[IBIS Ver]   3.2
[Comment Char]   |_char
[File Name]   sprm310.ibs
[File Rev]   1.0
[Date]   November 15, 2006
[Source]   From Ansoft Q3D ver 7.0 result.
[Notes]
[Disclaimer]
[Copyright]
[Component]   c2802ggm
[Manufacturer]   ti
[Package]
| variable   typ   min   max
R_pkg   2.43797e-001  1.95419e-001  3.27441e-001
L_pkg   3.68971n   2.87180n   5.33480n
C_pkg   0.700156p   0.378269p   1.23931p
[Pin]  signal_name   model_name   R_pin   L_pin   C_pin
B2   1   NC   2.35E-01   3.5513n   0.48473p
B1   2   NC   2.07E-01   3.0351n   0.467163p
C2   3   NC   2.47E-01   3.6211n   0.586473p
C3   4   NC   2.97E-01   4.5479n   0.708552p
C1   5   NC   2.19E-01   3.3047n   0.476389p
D2   6   NC   2.49E-01   3.6161n   0.555465p
D1   7   NC   2.15E-01   3.1776n   0.466284p
D3   8   NC   2.78E-01   4.1721n   0.675765p
E1   9   NC   2.16E-01   3.2216n   0.642896p
E2   10   NC   2.48E-01   3.6839n   0.861315p
E3   11   NC   2.90E-01   4.3193n   1.09313p
E4   12   NC   3.06E-01   4.8351n   1.23931p
E5   13   NC   3.27E-01   5.3348n   1.07834p
F1   14   NC   2.08E-01   3.0435n   0.550091p
F2   15   NC   2.37E-01   3.5019n   0.697553p
F3   16   NC   2.62E-01   4.1156n   1.04238p
F4   17   NC   2.93E-01   4.6685n   1.20271p
G4   18   NC   2.97E-01   4.7427n   1.03722p
G1   19   NC   2.03E-01   3.0288n   0.562932p
G2   20   NC   2.36E-01   3.4697n   0.651476p
G3   21   NC   2.72E-01   4.1098n   0.71232p
H1   22   NC   2.05E-01   3.0077n   0.489134p
H2   23   NC   2.38E-01   3.5337n   0.516547p
J1   24   NC   2.07E-01   3.0262n   0.418333p
K1   25   NC   2.15E-01   3.2729n   0.37954p
J2   26   NC   2.33E-01   3.5336n   0.483363p
K2   27   NC   2.03E-01   2.9784n   0.462757p
J3   28   NC   2.33E-01   3.4569n   0.577621p
H3   29   NC   2.71E-01   4.227n   0.695222p
K3   30   NC   1.95E-01   2.8906n   0.448812p
J4   31   NC   2.28E-01   3.374n   0.532016p
K4   32   NC   1.98E-01   2.8808n   0.454568p
H4   33   NC   2.65E-01   4.0698n   0.662835p
K5   34   NC   2.08E-01   3.1623n   0.638546p
J5   35   NC   2.46E-01   3.7519n   0.852293p
H5   36   NC   2.72E-01   4.2745n   1.07169p
G5   37   NC   2.97E-01   4.8506n   1.22295p
F5   38   NC   3.19E-01   5.2752n   1.05779p
K6   39   NC   2.07E-01   3.0553n   0.550089p
J6   40   NC   2.44E-01   3.6885n   0.755436p
H6   41   NC   2.74E-01   4.2729n   1.04565p
G6   42   NC   2.98E-01   4.6879n   1.20666p
G7   43   NC   3.08E-01   4.903n   1.03945p
K7   44   NC   2.10E-01   3.1053n   0.568618p
J7   45   NC   2.46E-01   3.6494n   0.659376p
H7   46   NC   2.88E-01   4.3538n   0.721025p
K8   47   NC   2.11E-01   3.1159n   0.491296p
J8   48   NC   2.47E-01   3.6522n   0.521398p
K9   49   NC   2.17E-01   3.2053n   0.425489p
K10   50   NC   2.14E-01   3.2751n   0.378399p
J9   51   NC   2.35E-01   3.5602n   0.485257p
J10   52   NC   2.07E-01   3.0498n   0.469529p
H9   53   NC   2.37E-01   3.5029n   0.580917p
H8   54   NC   2.75E-01   4.2366n   0.691548p
H10   55   NC   2.00E-01   2.9155n   0.45106p
G9   56   NC   2.36E-01   3.4315n   0.538278p
G10   57   NC   2.03E-01   2.922n   0.45761p
G8   58   NC   2.70E-01   4.1176n   0.665059p
F10   59   NC   2.11E-01   3.1329n   0.643673p
F9   60   NC   2.46E-01   3.6694n   0.861259p
F8   61   NC   2.69E-01   4.0897n   1.07509p
F7   62   NC   2.92E-01   4.5944n   1.22997p
F6   63   NC   3.16E-01   5.1049n   1.08148p
E10   64   NC   2.01E-01   2.9436n   0.545683p
E9   65   NC   2.33E-01   3.5044n   0.693789p
E8   66   NC   2.58E-01   3.8749n   1.01536p
E7   67   NC   2.92E-01   4.4776n   1.19334p
D7   68   NC   2.99E-01   4.6408n   1.05245p
D10   69   NC   2.03E-01   2.9695n   0.56445p
D9   70   NC   2.36E-01   3.5166n   0.653098p
D8   71   NC   2.72E-01   4.1552n   0.711568p
C10   72   NC   2.04E-01   2.9859n   0.489054p
C9   73   NC   2.39E-01   3.5077n   0.513094p
B10   74   NC   2.06E-01   3.0402n   0.420099p
A10   75   NC   2.15E-01   3.221n   0.378269p
B9   76   NC   2.32E-01   3.504n   0.484396p
A9   77   NC   2.04E-01   2.9488n   0.47194p
B8   78   NC   2.40E-01   3.5086n   0.579695p
C8   79   NC   2.78E-01   4.2509n   0.695399p
A8   80   NC   1.99E-01   2.9279n   0.450035p
B7   81   NC   2.32E-01   3.3433n   0.530971p
A7   82   NC   1.99E-01   2.9169n   0.453404p
C7   83   NC   2.68E-01   4.0651n   0.6638p
A6   84   NC   2.07E-01   3.0766n   0.639416p
B6   85   NC   2.40E-01   3.6014n   0.857213p
C6   86   NC   2.64E-01   4.0599n   1.07343p
D6   87   NC   2.86E-01   4.5728n   1.22123p
E6   88   NC   3.11E-01   5.1212n   1.06791p
A5   89   NC   1.97E-01   2.8718n   0.540838p
B5   90   NC   2.32E-01   3.4641n   0.743952p
C5   91   NC   2.56E-01   3.8795n   1.03595p
D5   92   NC   2.88E-01   4.5275n   1.1846p
D4   93   NC   2.95E-01   4.5747n   1.02693p
A4   94   NC   1.98E-01   2.9204n   0.560468p
B4   95   NC   2.32E-01   3.3841n   0.649932p
C4   96   NC   2.68E-01   3.9717n   0.711966p
A3   97   NC   2.03E-01   2.9754n   0.486969p
B3   98   NC   2.38E-01   3.5429n   0.511888p
A2   99   NC   2.03E-01   2.9877n   0.414459p
A1   100   NC   2.13E-01   3.1772n   0.378451p
[Define Package Model]  c2802
[Manufacturer]   ti
[OEM]   xyz
[Description]   c2802
[Number Of Pins]   100
[Pin Numbers]
B1   |   2
B2   |   1
C2   |   3
C3   |   4
C1   |   5
A1   |   100
B3   |   98
A2   |   99
C4   |   96
D3   |   8
D4   |   93
D2   |   6
D1   |   7
A3   |   97
D5   |   92
B4   |   95
E3   |   11
E2   |   10
E4   |   12
E5   |   13
E1   |   9
A4   |   94
E6   |   88
C5   |   91
F3   |   16
F2   |   15
F4   |   17
B5   |   90
F5   |   38
F6   |   63
F1   |   14
G4   |   18
A5   |   89
D6   |   87
F7   |   62
G5   |   37
G6   |   42
C6   |   86
B6   |   85
G7   |   43
E7   |   67
G1   |   19
A6   |   84
G2   |   20
C7   |   83
G3   |   21
F8   |   61
D7   |   68
H6   |   41
H5   |   36
G8   |   58
H7   |   46
B7   |   81
H8   |   54
E8   |   66
H4   |   33
D8   |   71
H1   |   22
A7   |   82
H2   |   23
C8   |   79
F9   |   60
H3   |   29
E9   |   65
D9   |   70
J5   |   35
H9   |   53
G9   |   56
J6   |   40
J8   |   48
J7   |   45
B8   |   78
J9   |   51
J4   |   31
J1   |   24
A8   |   80
J2   |   26
J3   |   28
C9   |   73
K5   |   34
K6   |   39
D10   |   69
F10   |   59
K7   |   44
E10   |   64
G10   |   57
H10   |   55
J10   |   52
K8   |   47
K4   |   32
B9   |   76
K9   |   49
K10   |   50
K1   |   25
A9   |   77
K3   |   30
C10   |   72
K2   |   27
B10   |   74
A10   |   75
[Model Data]
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[End Model Data]
[End Package Model]
|   Component BC3325CSFSHY
[Component]   BC3325CSFSHY
[Manufacturer]   Texas Instruments
[Package]
|  variable   typ   min   max
R_pkg   0   0   0
L_pkg   0   0   0
C_pkg   0   0   0
[Pin]   signal_name   model_name   R_pin   L_pin   C_pin
VSS   VSS   GND
VDDS   VDDS   POWER
PAD   PAD   BC3325CSFSHY
|   Component OC3325CS
[Component]   OC3325CS
[Manufacturer]   Texas Instruments
[Package]
|  variable   typ   min   max
R_pkg   0   0   0
L_pkg   0   0   0
C_pkg   0   0   0
[Pin]   signal_name   model_name   R_pin   L_pin   C_pin
VSS   VSS   GND
VDDS   VDDS   POWER
PAD   PAD   OC3325CS
|   Component IDH091_OUJ431
[Component]   IDH091_OUJ431
[Manufacturer]   Texas Instruments
[Package]
|  variable   typ   min   max
R_pkg   0   0   0
L_pkg   0   0   0
C_pkg   0   0   0
[Pin]   signal_name   model_name   R_pin   L_pin   C_pin
VSS   VSS   GND
VDDS   VDDS   POWER
PAD   PAD   IDH091_OUJ431
|   Component IC33SFSHYPD
[Component]   IC33SFSHYPD
[Manufacturer]   Texas Instruments
[Package]
|  variable   typ   min   max
R_pkg   0   0   0
L_pkg   0   0   0
C_pkg   0   0   0
[Pin]   signal_name   model_name   R_pin   L_pin   C_pin
VSS   VSS   GND
VDDS   VDDS   POWER
PAD   PAD   IC33SFSHYPD
[Model Selector] IC33SFSHYPD
PULLDOWN_ON_3P3_1  Cell operated at 3.3(nom)
|BUFFER OPERATING IN WEAK PULLDOWN MODE
PULLDOWN_OFF_3P3_1  Cell operated at 3.3(nom)
|   Component IC33SFSHY
[Component]   IC33SFSHY
[Manufacturer]   Texas Instruments
[Package]
|  variable   typ   min   max
R_pkg   0   0   0
L_pkg   0   0   0
C_pkg   0   0   0
[Pin]   signal_name   model_name   R_pin   L_pin   C_pin
VSS   VSS   GND
VDDS   VDDS   POWER
PAD   PAD   IC33SFSHY
|   Component BC3350ASHYPU
[Component]   BC3350ASHYPU
[Manufacturer]   Texas Instruments
[Package]
|  variable   typ   min   max
R_pkg   0   0   0
L_pkg   0   0   0
C_pkg   0   0   0
[Pin]   signal_name   model_name   R_pin   L_pin   C_pin
VSS   VSS   GND
VDDS   VDDS   POWER
PAD   PAD   BC3350ASHYPU
[Model Selector] BC3350ASHYPU
PULLUP_ON_3P3_2  Cell operated at 3.3(nom)
|BUFFER OPERATING IN WEAK PULLUP MODE
PULLUP_OFF_3P3_2  Cell operated at 3.3(nom)
|   Component BC3325CSHYPU
[Component]   BC3325CSHYPU
[Manufacturer]   Texas Instruments
[Package]
|  variable   typ   min   max
R_pkg   0   0   0
L_pkg   0   0   0
C_pkg   0   0   0
[Pin]   signal_name   model_name   R_pin   L_pin   C_pin
VSS   VSS   GND
VDDS   VDDS   POWER
PAD   PAD   BC3325CSHYPU
[Model Selector] BC3325CSHYPU
PULLUP_ON_3P3_3  Cell operated at 3.3(nom)
|BUFFER OPERATING IN WEAK PULLUP MODE
PULLUP_OFF_3P3_3  Cell operated at 3.3(nom)
|   Component OUJ431
[Component]   OUJ431
[Manufacturer]   Texas Instruments
[Package]
|  variable   typ   min   max
R_pkg   0   0   0
L_pkg   0   0   0
C_pkg   0   0   0
[Pin]   signal_name   model_name   R_pin   L_pin   C_pin
VSS   VSS   GND
VDDS   VDDS   POWER
PAD   PAD   OUJ431
|   Component IC33SFSHYPU
[Component]   IC33SFSHYPU
[Manufacturer]   Texas Instruments
[Package]
|  variable   typ   min   max
R_pkg   0   0   0
L_pkg   0   0   0
C_pkg   0   0   0
[Pin]   signal_name   model_name   R_pin   L_pin   C_pin
VSS   VSS   GND
VDDS   VDDS   POWER
PAD   PAD   IC33SFSHYPU
[Model Selector] IC33SFSHYPU
PULLUP_ON_3P3_4  Cell operated at 3.3(nom)
|BUFFER OPERATING IN WEAK PULLUP MODE
PULLUP_OFF_3P3_4  Cell operated at 3.3(nom)
|   Component BC3350BTODHYPU
[Component]   BC3350BTODHYPU
[Manufacturer]   Texas Instruments
[Package]
|  variable   typ   min   max
R_pkg   0   0   0
L_pkg   0   0   0
C_pkg   0   0   0
[Pin]   signal_name   model_name   R_pin   L_pin   C_pin
VSS   VSS   GND
VDDS   VDDS   POWER
PAD   PAD   BC3350BTODHYPU
| Models and submodels in the file (14): BC3325CSFSHY (I/O), OC3325CS (3-state), IDH091_OUJ431 (I/O), PULLDOWN_ON_3P3_1 (Input), PULLDOWN_OFF_3P3_1 (Input), IC33SFSHY (Input), PULLUP_ON_3P3_2 (I/O), PULLUP_OFF_3P3_2 (I/O), PULLUP_ON_3P3_3 (I/O), PULLUP_OFF_3P3_3 (I/O), OUJ431 (3-state), PULLUP_ON_3P3_4 (Input), PULLUP_OFF_3P3_4 (Input), BC3350BTODHYPU (I/O_open_drain)
